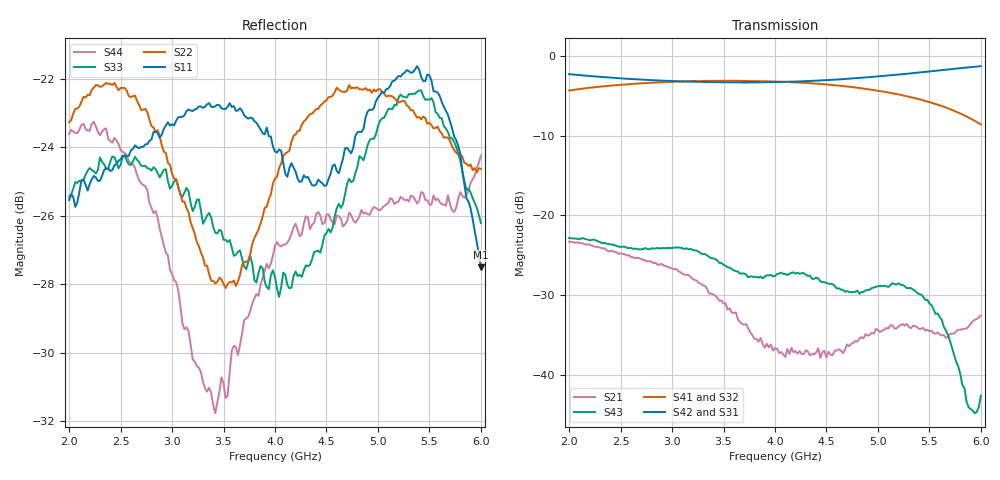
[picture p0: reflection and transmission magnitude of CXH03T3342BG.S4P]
!Agilent Technologies,E5071C,MY46418599,B.12.04
!Date: Mon Dec 16 02:30:10 2024
!Data & Calibration Information:
!Freq	S11:SOLT4(ON)	S12:SOLT4(ON)	S13:SOLT4(ON)	S14:SOLT4(ON)
!	S21:SOLT4(ON)	S22:SOLT4(ON)	S23:SOLT4(ON)	S24:SOLT4(ON)
!	S31:SOLT4(ON)	S32:SOLT4(ON)	S33:SOLT4(ON)	S34:SOLT4(ON)
!	S41:SOLT4(ON)	S42:SOLT4(ON)	S43:SOLT4(ON)	S44:SOLT4(ON)
!PortZ  Port1:50+j0  Port2:50+j0  Port3:50+j0  Port4:50+j0
!Above PortZ is port z conversion or system Z0 setting when saving the data.
!When reading, reference impedance value at option line is always used.
# Hz S dB R 50
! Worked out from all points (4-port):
!   201 points, 2 GHz to 6 GHz, reference 50 ohm
!   strongest paths, dB at 2 GHz, 3 GHz, 4 GHz, 5 GHz, 6 GHz:
!     S42: -2.3, -3.1, -3.3, -2.6, -1.3
!     S31: -2.3, -3.2, -3.3, -2.6, -1.3
!     S41: -4.3, -3.2, -3.2, -4.3, -8.6
!     S32: -4.3, -3.2, -3.2, -4.3, -8.5
!     S43: -22.8, -24.1, -27.6, -28.9, -42.6
!     S21: -23.3, -26.7, -36.7, -34.4, -32.6
!   lowest |S11| = -27.5 dB at 6 GHz (marker M1), VSWR 1.09, Z = 53.8 - j2.12 ohm
!   |S11| at or under -10 dB: start of sweep to end of sweep
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2e9  -25.54 143.3  -23.33 -8.7  -2.26 -63.4  -4.34 25.0
     -23.32 -8.4  -23.27 160.1  -4.32 26.1  -2.28 -63.8
     -2.26 -63.4  -4.33 26.1  -25.44 145.2  -22.83 -7.4
     -4.32 24.9  -2.27 -63.9  -22.84 -6.9  -23.61 164.9
3.42e9  -22.81 -165.2  -30.19 -95.0  -3.32 -93.6  -3.12 -4.4
        -30.09 -93.1  -27.98 -162.4  -3.09 -2.5  -3.29 -94.2
        -3.32 -93.5  -3.09 -2.3  -26.50 -169.3  -25.52 -95.5
        -3.11 -4.5  -3.27 -94.4  -25.51 -95.6  -31.76 -124.9
4.1e9  -24.78 -131.4  -37.69 -174.9  -3.29 -107.4  -3.28 -17.8
       -37.78 178.3  -24.18 -99.7  -3.24 -15.6  -3.26 -108.2
       -3.28 -107.3  -3.23 -15.4  -27.72 -113.8  -27.37 -165.5
       -3.25 -18.0  -3.24 -108.4  -27.35 -165.9  -26.84 -68.4
5.28e9  -21.75 -52.7  -34.25 71.2  -2.29 -134.9  -5.07 -44.2
        -33.62 71.9  -22.78 -71.8  -5.01 -40.8  -2.24 -135.9
        -2.28 -134.9  -5.01 -40.7  -22.55 -62.1  -28.77 77.4
        -5.04 -44.6  -2.22 -136.2  -29.14 76.0  -25.53 -45.4
5.62e9  -22.68 -45.4  -35.22 79.6  -1.83 -144.8  -6.29 -53.4
        -35.09 79.0  -23.59 -68.7  -6.23 -49.4  -1.78 -145.9
        -1.82 -144.8  -6.23 -49.2  -23.16 -71.9  -33.10 61.2
        -6.26 -53.7  -1.76 -146.1  -33.13 63.1  -25.67 -63.4
5.88e9  -25.59 -38.6  -34.03 94.1  -1.45 -153.2  -7.72 -60.8
        -33.97 96.1  -24.54 -68.7  -7.63 -56.2  -1.41 -154.3
        -1.47 -153.2  -7.66 -56.0  -25.20 -96.1  -44.67 89.2
        -7.72 -61.2  -1.41 -154.5  -44.09 80.7  -25.26 -93.5
6e9  -27.50 -27.9  -32.57 97.8  -1.31 -157.3  -8.61 -64.2
     -32.58 97.7  -24.63 -70.6  -8.50 -59.3  -1.26 -158.4
     -1.32 -157.3  -8.53 -59.1  -26.21 -111.9  -42.95 143.8
     -8.59 -64.6  -1.26 -158.6  -42.64 138.0  -24.24 -105.2
